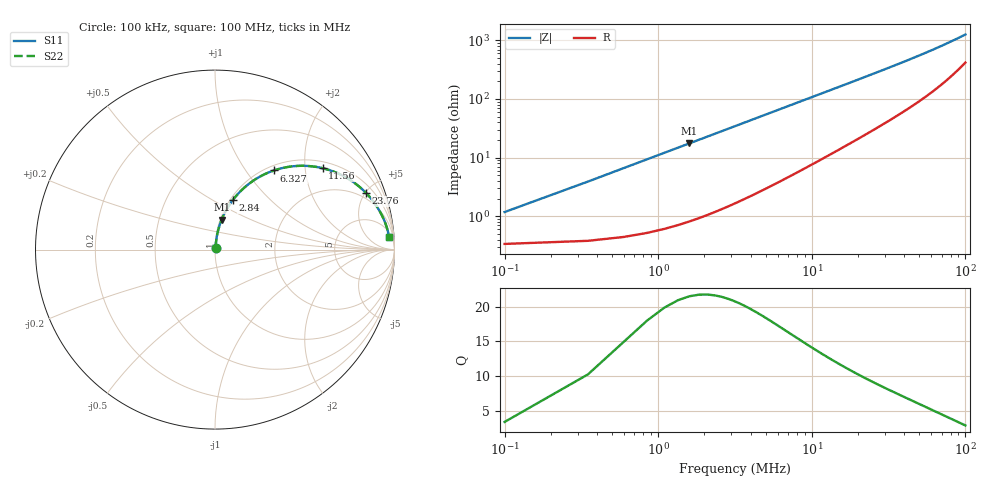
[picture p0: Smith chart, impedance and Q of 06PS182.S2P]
! Coilcraft 0603PS-182 Power Chip Inductor
! 19 February 2003
# MHZ S MA R 50
!Freq  MagS11  AngS11  MagS21  AngS21  MagS12  AngS12  MagS22  AngS22
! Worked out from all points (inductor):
!   403 points, 100 kHz to 100 MHz, reference 50 ohm
!   read as one part in series: L = 1.76 uH near 598.2 kHz
!   highest Q = 21.4 at 1.595 MHz (marker M1), where L = 1.74 uH
!   S11 on the Smith chart (normalised r, x): 100 kHz: 1.01, +0.02; 2.84 MHz: 1.03, +0.62; 6.327 MHz: 1.08, +1.36; 11.56 MHz: 1.19, +2.48; 23.76 MHz: 1.54, +5.07; 100 MHz: 9, +24
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0.1  0.01176 72.8  0.9966 -0.6  0.9966 -0.6  0.01176 72.8
0.3491  0.03894 82.2  0.9955 -2.2  0.9955 -2.2  0.03894 82.2
0.8473  0.09281 81.5  0.9905 -5.3  0.9905 -5.3  0.09281 81.5
1.0964  0.1193 80.3  0.9869 -6.8  0.9869 -6.8  0.1193 80.3
1.3455  0.1454 78.9  0.9825 -8.3  0.9825 -8.3  0.1454 78.9
1.5946  0.171 77.5  0.9773 -9.8  0.9773 -9.8  0.171 77.5
2.0928  0.2209 74.6  0.9652 -12.8  0.9652 -12.8  0.2209 74.6
2.8401  0.2918 70.3  0.9428 -16.9  0.9428 -16.9  0.2918 70.3
3.5874  0.3573 66.3  0.9165 -20.9  0.9165 -20.9  0.3573 66.3
4.3347  0.4172 62.4  0.8874 -24.6  0.8874 -24.6  0.4172 62.4
6.3275  0.5493 53.4  0.8039 -33.3  0.8039 -33.3  0.5493 53.4
8.5694  0.6567 45.3  0.7118 -40.9  0.7118 -40.9  0.6567 45.3
11.5586  0.7515 37.1  0.6055 -48.5  0.6055 -48.5  0.7515 37.1
14.0496  0.8033 32.1  0.5331 -53.2  0.5331 -53.2  0.8033 32.1
16.7897  0.8427 27.8  0.4683 -57.1  0.4683 -57.1  0.8427 27.8
20.028  0.8744 23.9  0.4073 -60.5  0.4073 -60.5  0.8744 23.9
23.7645  0.8991 20.5  0.3526 -63.4  0.3526 -63.4  0.8991 20.5
33.4794  0.9336 14.8  0.2581 -67.8  0.2581 -67.8  0.9336 14.8
50.1691  0.9568 9.8  0.1724 -70.7  0.1724 -70.7  0.9568 9.8
66.8588  0.966 7.1  0.126 -70.8  0.126 -70.8  0.966 7.1
83.5485  0.9701 5.4  0.09674 -69.3  0.09674 -69.3  0.9701 5.4
100  0.9719 4.2  0.07689 -66.5  0.07689 -66.5  0.9719 4.2
